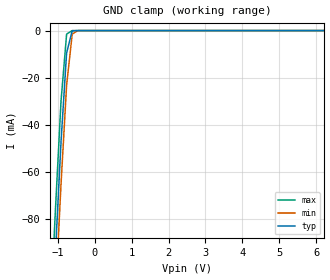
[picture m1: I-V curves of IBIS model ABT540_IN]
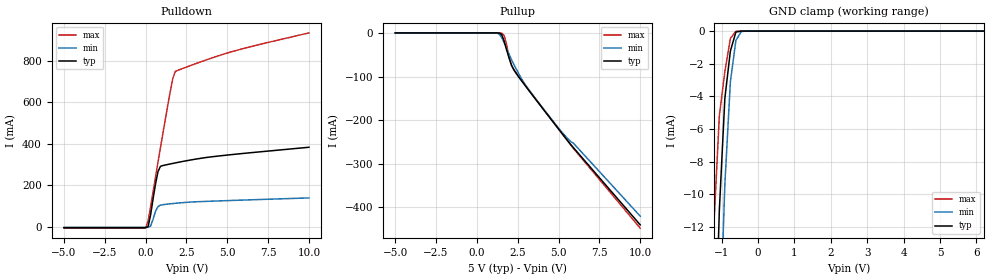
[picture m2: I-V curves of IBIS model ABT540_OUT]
|   TEXAS INSTRUMENTS INCORPORATED
|   Advanced Bus Interface Group
|   IBIS Model of SN74ABT540
|   OCTAL BUFFERS/DRIVERS WITH 3-STATE OUTPUTS
|   20-pin DW, DB, N & PW Package
[IBIS Ver]   2.1
[Comment char]  |_char
[File Name]   abt540.ibs
[File Rev]   1.1
[Date]   9/15/04
[Source]   File originated at Texas Instruments, Inc.
[Notes]   The following is a sample IBIS file for the ABT540.
   - This file may be incomplete or may not be fully compliant
   with the IBIS specification. It will be replaced with a
   version that is IBIS Revision 3.2 compliant and is complete
   and accurate. Please email all questions and comments to
   sllibis@ti.com.
   - FILE REV HISTORY
   - 1.1 Release IBIS file on 09/17/04
   - Power clamp data deleted as there is no power-clamp diode.
|   - All test data contained in this file are derived from
|   hspice(tm) simulations.
[Disclaimer] Property of Texas Instruments Incorporated
   Unauthorized reproduction and/or distribution is strictly
   prohibited.
   This product is protected under copyright law and trade
   secret law as an unpublished work.  Created 1998, (C)
   Copyright 1998, Texas Instruments Inc., All Rights Reserved
   These commodities are under U.S. Government distribution
   license control.  As such, they are not to be re-exported
   without prior approval of the U.S. Department of Commerce.
   Please be aware that in the absence of a written agreement
   to the contrary, Texas Instruments ("TI") assumes no
   liability for : (1) the accuracy of the IBIS models provided
   to your company;  (2) the proper functioning of these Models
   in your design system or for any resulting applications;
   or (3) infringement of patents, copyrights or intellectual
   property rights resulting from your use of these models.
   TI provides IBIS Models as a service to our customers and
   therefore reserves the right to limit distribution of the
   Models.
| Component ABT540_N 14-pin N
[Component]   ABT540_N
[Manufacturer]   Texas   Instruments,   Inc.
[Package]
|   typ   min   max
R_pkg   3.50E-02   2.40E-02   4.70E-02
L_pkg   2.40E-09   1.71E-09   3.25E-09
C_pkg   2.84E-13   1.66E-13   4.18E-13
[Pin] signal_name  model_name   R_pin   L_pin   C_pin
1   OE1_BAR   NC   4.10E-02   3.10E-09   4.10E-13
2   A1   ABT540_IN   4.00E-02   2.78E-09   3.63E-13
3   A2   ABT540_IN   2.90E-02   2.19E-09   2.60E-13
4   A3   ABT540_IN   2.50E-02   1.71E-09   1.66E-13
5   A4   ABT540_IN   2.50E-02   1.74E-09   1.91E-13
6   A5   ABT540_IN   2.40E-02   1.76E-09   1.93E-13
7   A6   ABT540_IN   2.40E-02   1.82E-09   1.74E-13
8   A7   ABT540_IN   2.80E-02   2.26E-09   2.65E-13
9   A8   ABT540_IN   4.50E-02   2.89E-09   3.68E-13
10   GND   GND   4.70E-02   3.25E-09   4.17E-13
11   Y8   ABT540_OUT   4.60E-02   3.24E-09   4.18E-13
12   Y7   ABT540_OUT   4.60E-02   2.96E-09   3.75E-13
13   Y6   ABT540_OUT   3.30E-02   2.33E-09   2.68E-13
14   Y5   ABT540_OUT   2.90E-02   1.92E-09   1.79E-13
15   Y4   ABT540_OUT   3.10E-02   1.93E-09   2.03E-13
16   Y3   ABT540_OUT   3.20E-02   1.92E-09   2.01E-13
17   Y2   ABT540_OUT   3.00E-02   1.83E-09   1.73E-13
18   Y1   ABT540_OUT   3.60E-02   2.32E-09   2.68E-13
19   OE2_BAR   NC   4.20E-02   2.87E-09   3.72E-13
20   VCC   POWER   4.20E-02   3.16E-09   4.14E-13
| Component ABT540_DB 14-pin DB
[Component]   ABT540_DB
[Manufacturer]   Texas   Instruments,   Inc.
[Package]
|   Mean.   Min.   Max.
R_pkg   0.04   0.035   0.051
L_pkg   3.495nH  3.035nH   4.314nH
C_pkg   0.42pF   0.346pF   0.502pF
[Pin]signal_name   model_name   R_pin   L_pin   C_pin
1   OE1_BAR   NC   0.049   4.31nH   0.502pF
2   A1   ABT540_IN   0.048   3.903nH   0.487pF
3   A2   ABT540_IN   0.035   3.189nH   0.396pF
4   A3   ABT540_IN   0.035   3.036nH   0.347pF
5   A4   ABT540_IN   0.035   3.035nH   0.367pF
6   A5   ABT540_IN   0.035   3.035nH   0.367pF
7   A6   ABT540_IN   0.035   3.036nH   0.347pF
8   A7   ABT540_IN   0.035   3.189nH   0.397pF
9   A8   ABT540_IN   0.047   3.899nH   0.488pF
10   GND   GND   0.051   4.314nH   0.5pF
11   Y8   ABT540_OUT   0.051   4.314nH   0.5pF
12   Y7   ABT540_OUT   0.047   3.899nH   0.488pF
13   Y6   ABT540_OUT   0.035   3.189nH   0.397pF
14   Y5   ABT540_OUT   0.035   3.036nH   0.346pF
15   Y4   ABT540_OUT   0.035   3.035nH   0.367pF
16   Y3   ABT540_OUT   0.035   3.035nH   0.367pF
17   Y2   ABT540_OUT   0.035   3.036nH   0.346pF
18   Y1   ABT540_OUT   0.035   3.189nH   0.397pF
19   OE2_BAR   NC   0.047   3.899nH   0.488pF
20   VCC   POWER   0.051   4.314nH   0.502pF
| Component ABT540_DW 14-pin DW
[Component]   ABT540_DW
[Manufacturer]   Texas   Instruments,   Inc.
[Package]
|   Mean.   Min.   Max.
R_pkg   0.038   0.033   0.045
L_pkg   5.012nH   4.11nH   6.349nH
C_pkg   0.717pF   0.53pF   0.868pF
[Pin]signal_name   model_name   R_pin   L_pin   C_pin
1   OE1_BAR   NC   0.042   6.336nH   0.865pF
2   A1   ABT540_IN   0.043   5.542nH   0.867pF
3   A2   ABT540_IN   0.034   4.714nH   0.732pF
4   A3   ABT540_IN   0.034   4.377nH   0.591pF
5   A4   ABT540_IN   0.036   4.13nH   0.533pF
6   A5   ABT540_IN   0.035   4.111nH   0.53pF
7   A6   ABT540_IN   0.034   4.284nH   0.583pF
8   A7   ABT540_IN   0.034   4.634nH   0.726pF
9   A8   ABT540_IN   0.04   5.518nH   0.865pF
10   GND   GND   0.043   6.349nH   0.866pF
11   Y8   ABT540_OUT   0.041   6.281nH   0.861pF
12   Y7   ABT540_OUT   0.045   5.561nH   0.868pF
13   Y6   ABT540_OUT   0.033   4.778nH   0.742pF
14   Y5   ABT540_OUT   0.035   4.414nH   0.596pF
15   Y4   ABT540_OUT   0.035   4.11nH   0.533pF
16   Y3   ABT540_OUT   0.036   4.13nH   0.533pF
17   Y2   ABT540_OUT   0.034   4.377nH   0.591pF
18   Y1   ABT540_OUT   0.034   4.714nH   0.731pF
19   OE2_BAR   NC   0.043   5.569nH   0.868pF
20   VCC   POWER   0.042   6.308nH   0.864pF
| Component ABT540_PW 20-pin PW
[Component]   ABT540_PW
[Manufacturer]   Texas Instruments, Inc.
[Package]
|   typ   min   max
R_pkg   5.000e-02   4.200e-02   6.000e-02
L_pkg   2.802e-09   2.248e-09   3.553e-09
C_pkg   3.170e-13   2.020e-13   4.430e-13
[Pin]   signal_name   model_name   R_pin   L_pin   C_pin
1   OE1_BAR   NC   5.500e-02   3.461e-09   4.400e-13
2   A1   ABT540_IN   5.500e-02   3.150e-09   4.010e-13
3   A2   ABT540_IN   4.200e-02   2.619e-09   3.020e-13
4   A3   ABT540_IN   4.500e-02   2.273e-09   2.020e-13
5   A4   ABT540_IN   4.500e-02   2.248e-09   2.240e-13
6   A5   ABT540_IN   4.500e-02   2.273e-09   2.260e-13
7   A6   ABT540_IN   4.400e-02   2.323e-09   2.050e-13
8   A7   ABT540_IN   4.600e-02   2.704e-09   3.070e-13
9   A8   ABT540_IN   6.000e-02   3.265e-09   4.110e-13
10   GND   GND   5.700e-02   3.506e-09   4.360e-13
11   Y8   ABT540_OUT   5.800e-02   3.553e-09   4.370e-13
12   Y7   ABT540_OUT   5.800e-02   3.193e-09   4.050e-13
13   Y6   ABT540_OUT   4.200e-02   2.704e-09   3.110e-13
14   Y5   ABT540_OUT   4.600e-02   2.392e-09   2.100e-13
15   Y4   ABT540_OUT   4.700e-02   2.334e-09   2.290e-13
16   Y3   ABT540_OUT   4.700e-02   2.300e-09   2.270e-13
17   Y2   ABT540_OUT   4.700e-02   2.349e-09   2.070e-13
18   Y1   ABT540_OUT   4.500e-02   2.677e-09   3.060e-13
19   OE2_BAR   NC   6.000e-02   3.235e-09   4.060e-13
20   VCC   POWER   5.600e-02   3.487e-09   4.430e-13
| Models and submodels in the file (2): ABT540_IN (Input), ABT540_OUT (3-state)
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| Model ABT540_IN
[Model]   ABT540_IN
Model_type   Input
Polarity   Inverting
Vinh = 2.0
Vinl = 0.8
|   typ   min   max
C_comp   3pF   NA   NA
[Temperature Range]   25   -40   85
[Voltage Range]   5.0   4.5   5.5
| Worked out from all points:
|   GND clamp passes 1 mA (typ) near -0.62 V on its own axis
[gnd_clamp]
|   Voltage   I(typ)   I(min)   I(max)
-5V       -1.478A    -1.494A    -1.462A
-1.212V   -144.4mA   -162.9mA   -126.1mA
-1.061V   -94.44mA   -113mA     -76.13mA
-909.5mV  -47.24mA   -65.19mA   -29.92mA
-758mV    -9.43mA    -23.13mA   -1.504mA
-606.5mV  -117.8uA   -1.472mA   -3.356uA
-455mV    -585.3nA   -17.02uA   -6.291nA
9.998V    2nA        2.016nA    2nA
| Model ABT540_OUT
[Model]   ABT540_OUT
Model_type   3-state
Polarity   Non-Inverting
Enable   Active-Low
|   typ   min   max
C_comp   8pF   NA   NA
[Temperature Range]   25   -40   85
[Voltage range]   5.0   4.5   5.5
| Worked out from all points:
|   slope of the pulldown table from 0 to 0.75 V, typ, clamps not added: 2.82 ohm
|   GND clamp passes 1 mA (typ) near -0.73 V on its own axis
[Pullup]   | Vtable = Vcc - Voutput
|   Voltage   I(typ)   I(min)   I(max)
-5V       -414.4pA   -390pA     -440.3pA
1.06V     -1.563uA   -30.66uA   -4.395nA
1.363V    -352.1uA   -2.539mA   -16.23uA
1.514V    -3.928mA   -10.43mA   -389.4uA
1.666V    -18.18mA   -22.33mA   -6.027mA
1.969V    -57.59mA   -48.94mA   -54.48mA
2.12V     -74.03mA   -61.4mA    -75.16mA
2.424V    -93.82mA   -83.85mA   -92.51mA
3.181V    -131.9mA   -130.4mA   -130.7mA
5.151V    -227.6mA   -225.1mA   -227.5mA
5.908V    -263mA     -252.8mA   -264.6mA
9.998V    -440mA     -420mA     -447.6mA
[pulldown]
|   Voltage   I(typ)   I(min)   I(max)
-5V       -2.666mA   -1.663mA   -5.255mA
-500uV    -2.551mA   -1.598mA   -4.361mA
151mV     1.734mA    -1.187mA   29.02mA
302.5mV   57mA       4.614mA    95.88mA
605.5mV   206.4mA    75.27mA    240.2mA
757mV     266.5mA    98.44mA    311.7mA
908.5mV   291.9mA    105.4mA    381.6mA
1.514V    303.4mA    111.8mA    653.9mA
1.666V    305.9mA    113mA      714.4mA
1.817V    308.3mA    114.2mA    747.8mA
5.151V    347.3mA    127.6mA    840mA
9.998V    383.6mA    140.1mA    933.2mA
[gnd_clamp]
|   Voltage   I(typ)   I(min)   I(max)
-5V       -913.9mA   -859.6mA   -921.4mA
-1.364V   -35.15mA   -47.25mA   -23.88mA
-1.212V   -21.9mA    -31.83mA   -11.94mA
-1.061V   -10.96mA   -19.45mA   -5.173mA
-909.5mV  -4.105mA   -9.363mA   -2.473mA
-758mV    -1.216mA   -3.099mA   -454.3uA
-606.5mV  -59.78uA   -566.1uA   -5.882uA
-455mV    -753.1nA   -24.32uA   -127.8nA
-303.5mV  -55.52nA   -435.8nA   -73.91nA
9.998V    5.956nA    6.238nA    5.935nA
[ramp]
| variable   typ   min   max
dV/dt_r   1.7889E+00/8.8105E-10  1.4981E+00/1.5820E-09  2.1078E+00/1.6173E-09
dV/dt_f   2.7781E+00/1.2540E-09  2.3328E+00/1.4824E-09  3.1084E+00/8.5995E-10
